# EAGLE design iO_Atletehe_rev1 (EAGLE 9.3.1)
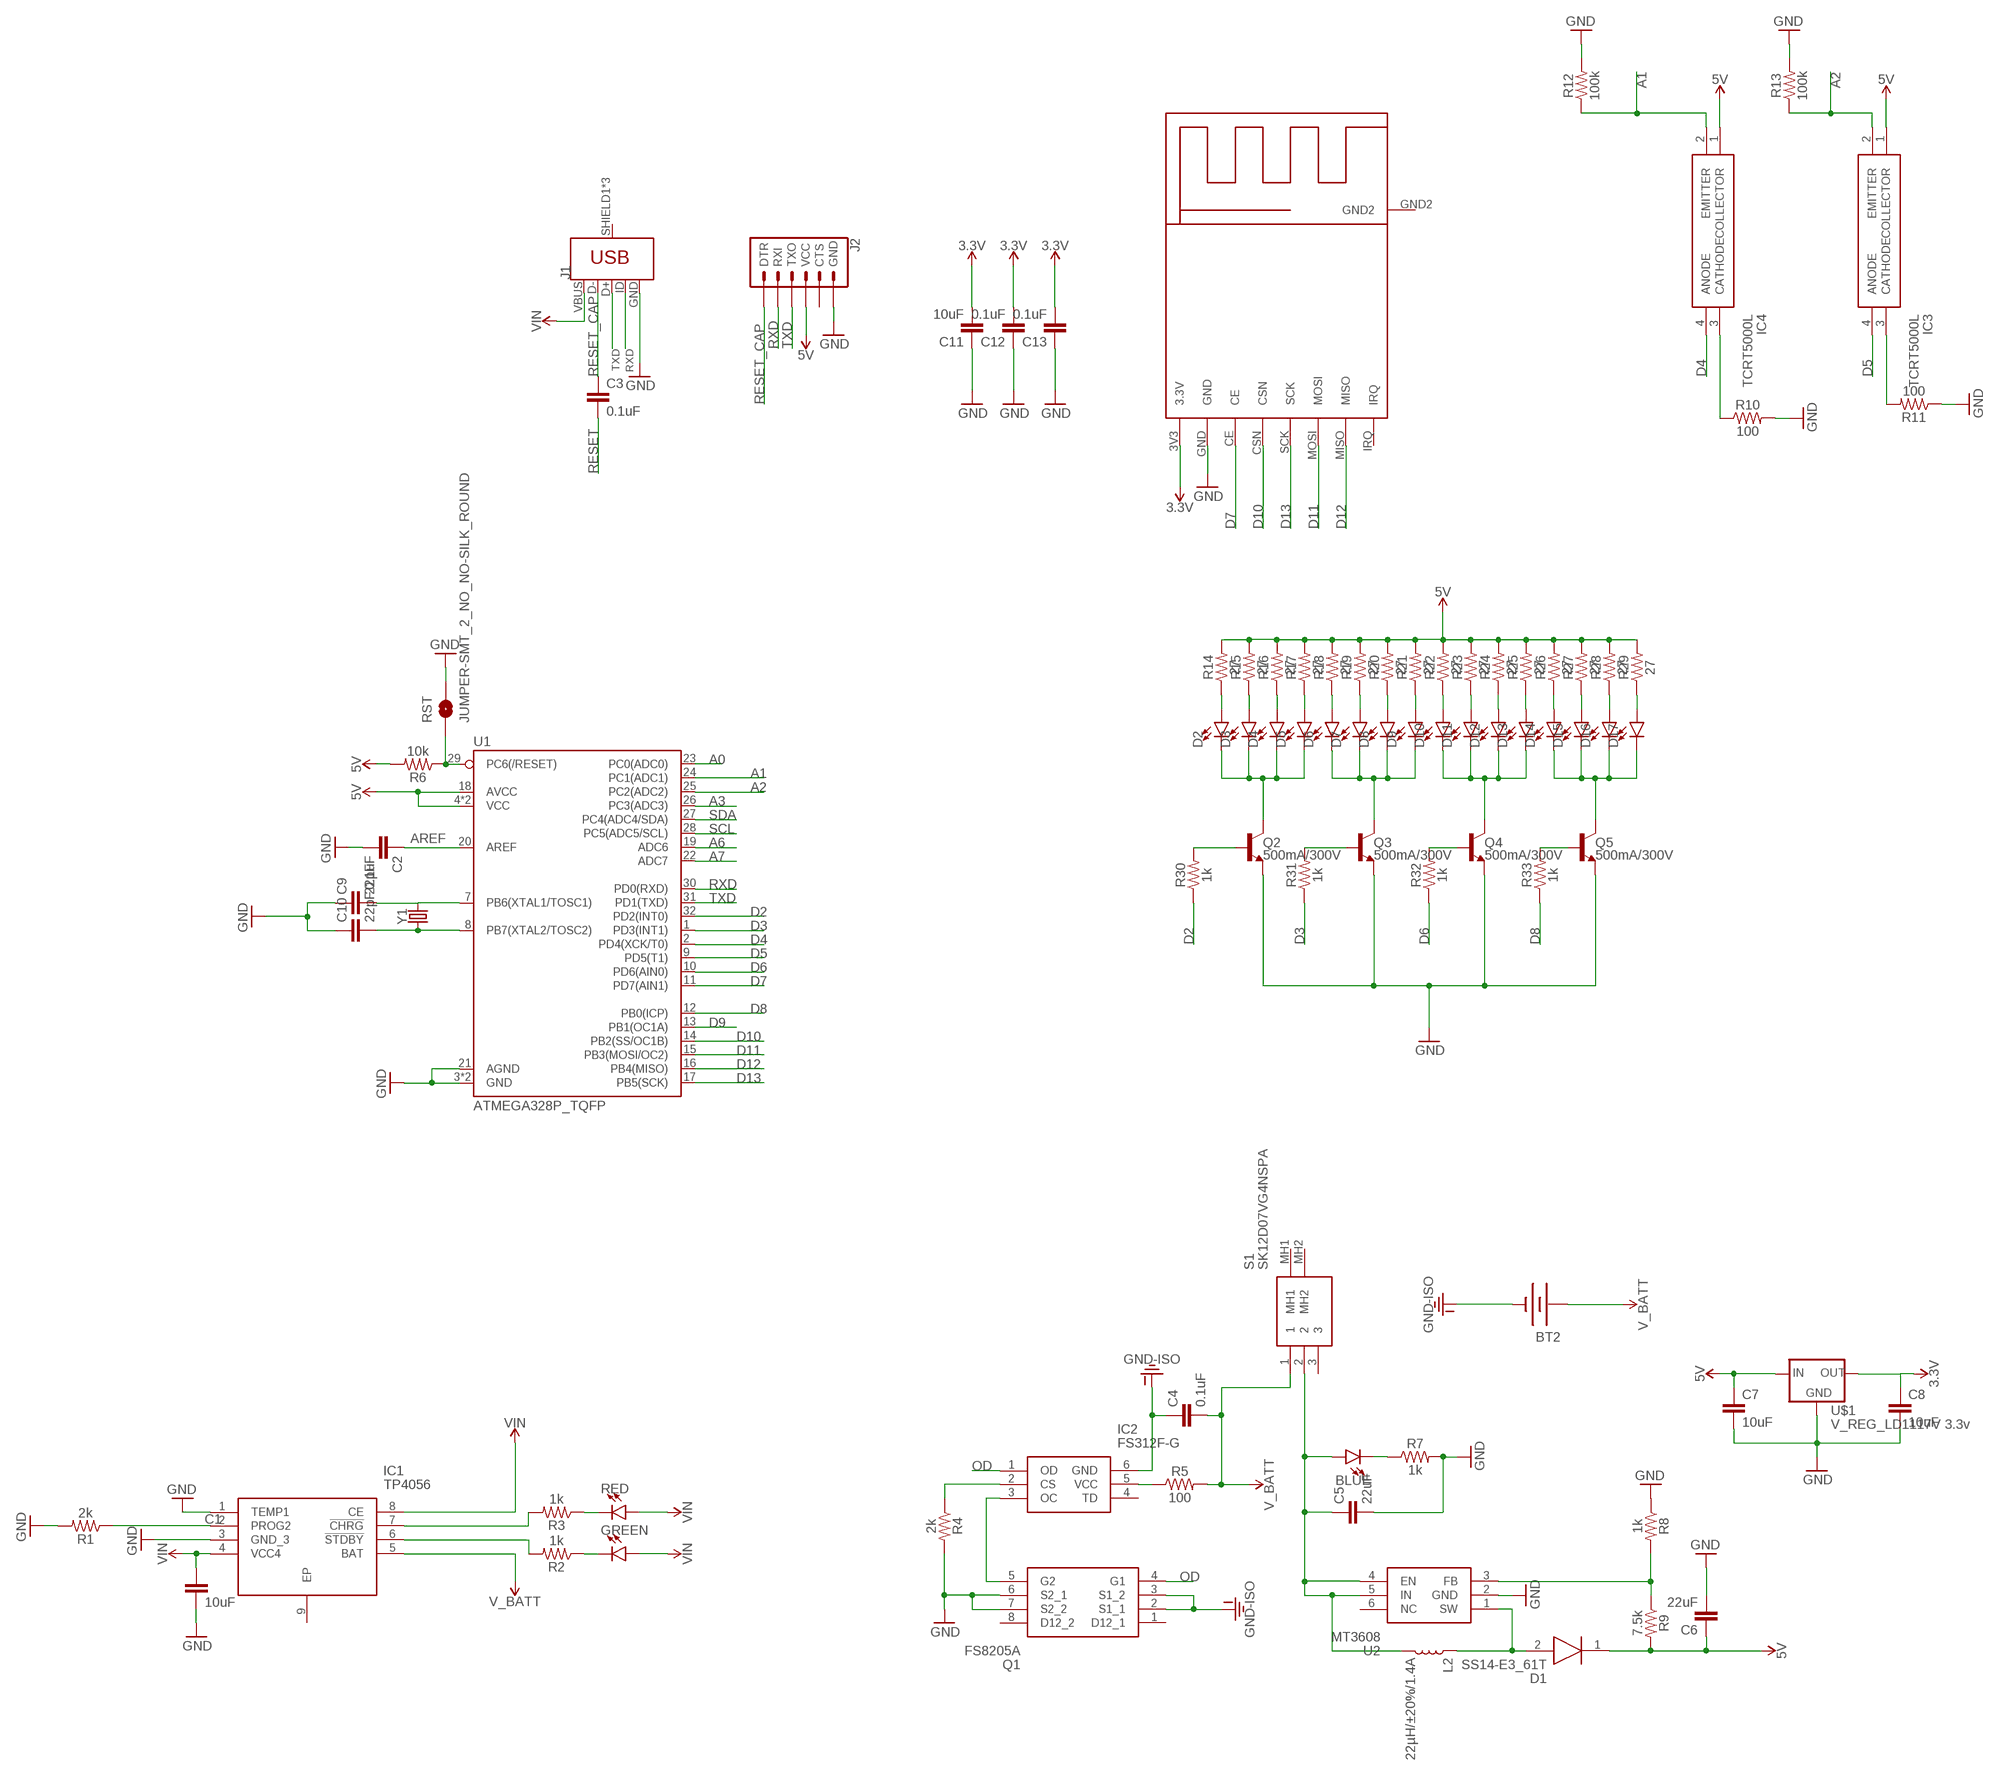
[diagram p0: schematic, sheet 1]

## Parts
BLUE  LED0603  [LED-0603]
BT2  BATTERY1100  [LIPO-1100MAH]
C1  10uF  10UF-0603-6.3V-20%  [0603]
C2  0.1uF  0.1UF-0603-25V-5%  [0603]
C3  0.1uF  0.1UF-0603-25V-5%  [0603]
C4  0.1uF  0.1UF-0603-25V-5%  [0603]
C5  22uF  10UF-0603-6.3V-20%  [0603]
C6  22uF  10UF-0603-6.3V-20%  [0603]
C7  10uF  10UF-0603-6.3V-20%  [0603]
C8  10uF  10UF-0603-6.3V-20%  [0603]
C9  22pF  22PF-0603-50V-5%  [0603]
C10  22pF  22PF-0603-50V-5%  [0603]
C11  10uF  10UF-0603-6.3V-20%  [0603]
C12  0.1uF  0.1UF-0603-25V-5%  [0603]
C13  0.1uF  0.1UF-0603-25V-5%  [0603]
D1  SS14-E3_61T  [DIOM5127X229N]
D2  LED5MM  [LED_5MM]
D3  LED5MM  [LED_5MM]
D4  LED5MM  [LED_5MM]
D5  LED5MM  [LED_5MM]
D6  LED5MM  [LED_5MM]
D7  LED5MM  [LED_5MM]
D8  LED5MM  [LED_5MM]
D9  LED5MM  [LED_5MM]
D10  LED5MM  [LED_5MM]
D11  LED5MM  [LED_5MM]
D12  LED5MM  [LED_5MM]
D13  LED5MM  [LED_5MM]
D14  LED5MM  [LED_5MM]
D15  LED5MM  [LED_5MM]
D16  LED5MM  [LED_5MM]
D17  LED5MM  [LED_5MM]
GREEN  LED0603  [LED-0603]
IC1  TP4056  [SOIC127P600X175-9N]
IC2  FS312F-G  [SOT95P280X145-6N]
IC3  TCRT5000L  [TCRT5000L]
IC4  TCRT5000L  [TCRT5000L]
J1  USB_MICRO-B_FEMALE-SMT  [USB-B-MICRO-SMD]
J2  6_PIN_SERIAL_TARGETPTH-KIT  [1X06-KIT]
L2  22µH/±20%/1.4A  INDUCTOR-SRN6045-33UH  [SRN6045]
Q1  FS8205A  [SOP65P640X120-8N]
Q2  500mA/300V  TRANS_NPN-MMBTA42  [SOT23-3]
Q3  500mA/300V  TRANS_NPN-MMBTA42  [SOT23-3]
Q4  500mA/300V  TRANS_NPN-MMBTA42  [SOT23-3]
Q5  500mA/300V  TRANS_NPN-MMBTA42  [SOT23-3]
R1  2k  10KOHM-0603-1/10W-1%  [0603]
R2  1k  10KOHM-0603-1/10W-1%  [0603]
R3  1k  10KOHM-0603-1/10W-1%  [0603]
R4  2k  10KOHM-0603-1/10W-1%  [0603]
R5  100  10KOHM-0603-1/10W-1%  [0603]
R6  10k  10KOHM-0603-1/10W-1%  [0603]
R7  1k  10KOHM-0603-1/10W-1%  [0603]
R8  1k  10KOHM-0603-1/10W-1%  [0603]
R9  7.5k  10KOHM-0603-1/10W-1%  [0603]
R10  100  10KOHM-0603-1/10W-1%  [0603]
R11  100  10KOHM-0603-1/10W-1%  [0603]
R12  100k  10KOHM-0603-1/10W-1%  [0603]
R13  100k  10KOHM-0603-1/10W-1%  [0603]
R14  27  27OHM-0603-1/10W-1%  [0603]
R15  27  27OHM-0603-1/10W-1%  [0603]
R16  27  27OHM-0603-1/10W-1%  [0603]
R17  27  27OHM-0603-1/10W-1%  [0603]
R18  27  27OHM-0603-1/10W-1%  [0603]
R19  27  27OHM-0603-1/10W-1%  [0603]
R20  27  27OHM-0603-1/10W-1%  [0603]
R21  27  27OHM-0603-1/10W-1%  [0603]
R22  27  27OHM-0603-1/10W-1%  [0603]
R23  27  27OHM-0603-1/10W-1%  [0603]
R24  27  27OHM-0603-1/10W-1%  [0603]
R25  27  27OHM-0603-1/10W-1%  [0603]
R26  27  27OHM-0603-1/10W-1%  [0603]
R27  27  27OHM-0603-1/10W-1%  [0603]
R28  27  27OHM-0603-1/10W-1%  [0603]
R29  27  27OHM-0603-1/10W-1%  [0603]
R30  1k  1KOHM-0603-1/10W-1%  [0603]
R31  1k  1KOHM-0603-1/10W-1%  [0603]
R32  1k  1KOHM-0603-1/10W-1%  [0603]
R33  1k  1KOHM-0603-1/10W-1%  [0603]
RED  LED0603  [LED-0603]
RST  JUMPER-SMT_2_NO_NO-SILK_ROUND  [SMT-JUMPER_2_NO_NO-SILK_ROUND]
S1  SK12D07VG4NSPA  [SK12D07VG4NSPA]
U1  ATMEGA328P_TQFP  [TQFP32-08]
U2  MT3608  [SOT95P280X145-6N]
U$1  V_REG_LD1117V 3.3v  V_REG_LD1117VXXLD1117-SMD  [SOT223]
U$2  NRF24MINI  [NRF24MINI]
Y1  CRYSTALSMD-HC49UP  [HC49UP]

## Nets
3.3V: C8.1 C11.2 C12.2 C13.2 U$1.2(OUT) U$2.3V3(3.3V)
5V: C6.1 C7.1 D1.1(K) IC3.1(COLLECTOR) IC4.1(COLLECTOR) J2.4(VCC) R6.2 R9.2 R14.2 R15.2 R16.2 R17.2 R18.2 R19.2 R20.2 R21.2 R22.2 R23.2 R24.2 R25.2 R26.2 R27.2 R28.2 R29.2 U1.4(VCC) U1.6(VCC) U1.18(AVCC) U$1.3(IN)
A0: U1.23(PC0(ADC0))
A1: IC4.2(EMITTER) R12.1 U1.24(PC1(ADC1))
A2: IC3.2(EMITTER) R13.1 U1.25(PC2(ADC2))
A3: U1.26(PC3(ADC3))
A6: U1.19(ADC6)
A7: U1.22(ADC7)
AREF: C2.1 U1.20(AREF)
D2: R30.1 U1.32(PD2(INT0))
D3: R31.1 U1.1(PD3(INT1))
D4: IC4.4(ANODE) U1.2(PD4(XCK/T0))
D5: IC3.4(ANODE) U1.9(PD5(T1))
D6: R32.1 U1.10(PD6(AIN0))
D7: U1.11(PD7(AIN1)) U$2.CE
D8: R33.1 U1.12(PB0(ICP))
D9: U1.13(PB1(OC1A))
D10: U1.14(PB2(SS/OC1B)) U$2.CSN
D11: U1.15(PB3(MOSI/OC2)) U$2.MOSI
D12: U1.16(PB4(MISO)) U$2.MISO
D13: U1.17(PB5(SCK)) U$2.SCK
GND [power]: C1.2 C2.2 C5.2 C6.2 C7.2 C8.2 C9.1 C10.1 C11.1 C12.1 C13.1 IC1.1(TEMP1) IC1.3(GND_3) J1.GND J2.6(GND) Q1.6(S2_1) Q1.7(S2_2) Q2.2(E) Q3.2(E) Q4.2(E) Q5.2(E) R1.2 R4.2 R7.2 R8.1 R10.2 R11.1 R12.2 R13.2 RST.2 U1.3(GND) U1.5(GND) U1.21(AGND) U2.2(GND) U$1.1(GND) U$2.GND
GND-ISO: BT2.- C4.1 IC2.6(GND) Q1.2(S1_1) Q1.3(S1_2)
N$1: IC2.3(OC) Q1.5(G2)
N$2: BLUE.C R7.1
N$3: IC1.2(PROG2) R1.1
N$4: GREEN.C R2.1
N$5: R3.1 RED.C
N$6: IC1.6(!STDBY) R2.2
N$7: IC1.7(!CHRG) R3.2
N$8: IC2.2(CS) R4.1
N$9: IC2.5(VCC) R5.1
N$10: C9.2 U1.7(PB6(XTAL1/TOSC1)) Y1.2
N$11: C10.2 U1.8(PB7(XTAL2/TOSC2)) Y1.1
N$12: D1.2(A) L2.1 U2.1(SW)
N$13: R8.2 R9.1 U2.3(FB)
N$14: BLUE.A C5.1 L2.2 S1.2 U2.4(EN) U2.5(IN)
N$15: IC4.3(CATHODE) R10.1
N$16: D2.A R14.1
N$17: IC3.3(CATHODE) R11.2
N$18: D3.A R15.1
N$19: D4.A R16.1
N$20: D5.A R17.1
N$21: D6.A R18.1
N$22: D7.A R19.1
N$23: D8.A R20.1
N$24: D9.A R21.1
N$25: D10.A R22.1
N$26: D11.A R23.1
N$27: D14.A R26.1
N$28: D13.A R25.1
N$29: D12.A R24.1
N$30: D15.A R27.1
N$31: D16.A R28.1
N$32: D17.A R29.1
N$34: D2.K(C) D3.K(C) D4.K(C) D5.K(C) Q2.3(C)
N$35: D6.K(C) D7.K(C) D8.K(C) D9.K(C) Q3.3(C)
N$36: D10.K(C) D11.K(C) D12.K(C) D13.K(C) Q4.3(C)
N$37: D14.K(C) D15.K(C) D16.K(C) D17.K(C) Q5.3(C)
N$38: Q2.1(B) R30.2
N$39: Q3.1(B) R31.2
N$40: Q4.1(B) R32.2
N$41: Q5.1(B) R33.2
OD: IC2.1(OD) Q1.4(G1)
RESET: C3.2 R6.1 RST.1 U1.29(PC6(/RESET))
RESET_CAP: C3.1 J1.D- J2.1(DTR)
RXD: J1.ID J2.2(RXI) U1.30(PD0(RXD))
SCL: U1.28(PC5(ADC5/SCL))
SDA: U1.27(PC4(ADC4/SDA))
TXD: J1.D+ J2.3(TXO) U1.31(PD1(TXD))
V_BATT: BT2.+ C4.2 IC1.5(BAT) R5.2 S1.1
VIN: C1.1 GREEN.A IC1.4(VCC4) IC1.8(CE) J1.VBUS RED.A
Unconnected: IC1.9(EP) IC2.4(TD) J1.SHIELD1(SHIELD) J1.SHIELD2(SHIELD) J1.SHIELD3(SHIELD) J2.5(CTS) Q1.1(D12_1) Q1.8(D12_2) S1.3 S1.MH1 S1.MH2 U2.6(NC) U$2.GND2 U$2.IRQ

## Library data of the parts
BLUE D2-D17 GREEN RED = SparkFun-LED:LED: LED (Generic)
BT2 = SparkFun-Retired:BATTERY: Battery - Single Cell
C1 C7 C8 C11 = SparkFun-Capacitors:10UF: 10.0µF ceramic capacitors; PROD_ID: CAP-11015
C2-C4 C12 C13 = SparkFun-Capacitors:0.1UF: 0.1µF ceramic capacitors; PROD_ID: CAP-08604
C5 C6 = SparkFun-Capacitors:10UF: 10.0µF ceramic capacitors; PROD_ID: CAP-11015; VALUE: 10uF
C9 C10 = SparkFun-Capacitors:22PF: 22pF ceramic capacitors; PROD_ID: CAP-07876
D1 = SS14-E3_61T:SS14-E3_61T: Schottky Diode 1A 40V 0.5Vf DO-214AC Vishay SS14-E3/61T, SMT Schottky Diode, 40V 1A, 2-Pin DO-214AC; ALLIED_NUMBER: 70217666; ALLIED_PRICE-STOCK: https://www.alliedelec.com/general-semiconductor-vishay-ss14-e3-61t/70217666/; DESCRIPTION: Schottky Diode 1A 40V 0.5Vf DO-214AC Vishay SS14-E3/61T, SMT Schottky Diode, 40V 1A, 2-Pin DO-214AC; HEIGHT: 2.29mm; MANUFACTURER_NAME: Vishay; MANUFACTURER_PART_NUMBER: SS14-E3/61T; MOUSER_PART_NUMBER: 625-SS14-E3; MOUSER_PRICE-STOCK: https://www.mouser.com/Search/Refine.aspx?Keyword=625-SS14-E3; RS_PART_NUMBER: 6387915P; RS_PRICE-STOCK: http://uk.rs-online.com/web/p/products/6387915P
IC1 = TP4056:TP4056: 1A Standalone Linear Li-lon Battery Charger, SOP-8 Source: Datasheet; DESCRIPTION: 1A Standalone Linear Li-lon Battery Charger, SOP-8; HEIGHT: 1.75mm; MANUFACTURER_NAME: NanJing Top Power; MANUFACTURER_PART_NUMBER: TP4056
IC2 = FS312F-G:FS312F-G: One Cell Lithium-ion/Polymer Battery Protection IC Source: Datasheet; DESCRIPTION: One Cell Lithium-ion/Polymer Battery Protection IC; HEIGHT: 1.45mm; MANUFACTURER_NAME: Fortune Semiconductor Corporation; MANUFACTURER_PART_NUMBER: FS312F-G
IC3 IC4 = TCRT5000L:TCRT5000L: Photointerrupter Reflective Phototransi Vishay TCRT5000L PCB Through Hole Reflective Optical Sensor, Transistor Output 2, Leaded Package Source: Datasheet; ALLIED_NUMBER: 70617350; ALLIED_PRICE-STOCK: http://www.alliedelec.com/siliconix-vishay-tcrt5000l/70617350/; DESCRIPTION: Photointerrupter Reflective Phototransi Vishay TCRT5000L PCB Through Hole Reflective Optical Sensor, Transistor Output 2, Leaded Package; HEIGHT: mm; MANUFACTURER_NAME: Vishay; MANUFACTURER_PART_NUMBER: TCRT5000L; MOUSER_PART_NUMBER: 782-TCRT5000L; MOUSER_PRICE-STOCK: https://www.mouser.com/Search/Refine.aspx?Keyword=782-TCRT5000L; RS_PART_NUMBER: 1451738; RS_PRICE-STOCK: http://uk.rs-online.com/web/p/products/1451738
J1 = SparkFun-Connectors:USB_MICRO-B: USB Type Micro-B Connector Male/female and PTH/SMT variants SparkFun Products: SparkFun microB USB Breakout SparkFun USB microB Plug Breakout SparkFun ESP8266 Thing; PROD_ID: CONN-11752
J2 = SparkFun-Connectors:6_PIN_SERIAL_TARGET: 6-pin header connection for use with the "FTDI BASIC" pinout - TARGET SIDE. Also known as "Arduino Serial Program Header". It is used to mate with our FTDI Basic serial programmers using the Arduino IDE. Note, this device has "TARGET" in the name. It is intended to be used on a design that contains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
L2 = SparkFun-Coils:INDUCTOR: Inductors; PROD_ID: NDUC-11627; VALUE: 33µH/±20%/1.4A
Q1 = FS8205A:FS8205A: dual n-channel enhancement mode power MOFSET Source: Datasheet; DESCRIPTION: dual n-channel enhancement mode power MOFSET; HEIGHT: 1.2mm; MANUFACTURER_NAME: SII Semiconductor; MANUFACTURER_PART_NUMBER: FS8205A
Q2-Q5 = SparkFun-DiscreteSemi:TRANS_NPN: NPN transistor Current controlled devices typically used to amplify current or used as a switch. BC547 - COM-08928 (TO-92 45V 100mA) (1.Collector 2.Base 3.Emitter) 2N3904 - COM-00521 (TO-92 40V 200mA) (1.Emitter 2.Base 3.Collector) P2N2222A - COM-12852 (TO-92 40V 600mA) (1.Collector 2.Base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; PROD_ID: TRANS-09116
R1-R5 R7-R13 = SparkFun-Resistors:10KOHM: 10kΩ resistor; PROD_ID: RES-00824; VALUE: 10k
R6 = SparkFun-Resistors:10KOHM: 10kΩ resistor; PROD_ID: RES-00824
R14-R29 = SparkFun-Resistors:27OHM: 27Ω resistor; PROD_ID: RES-09334
R30-R33 = SparkFun-Resistors:1KOHM: 1kΩ resistor; PROD_ID: RES-07856
RST = SparkFun-Jumpers:JUMPER-SMT_2_NO: Normally open jumper
S1 = SK12D07VG4NSPA:SK12D07VG4NSPA: Slide Switches Miniature Slide Switch Source: Datasheet; DESCRIPTION: Slide Switches Miniature Slide Switch; HEIGHT: 4.7mm; MANUFACTURER_NAME: C & K COMPONENTS; MANUFACTURER_PART_NUMBER: SK12D07VG4NSPA; MOUSER_PART_NUMBER: 611-SK12D07VG4NSPA; MOUSER_PRICE-STOCK: https://www.mouser.com/Search/Refine.aspx?Keyword=611-SK12D07VG4NSPA
U1 = SparkFun-IC-Microcontroller:ATMEGA328P_TQFP: Popular 328P in QFP Storefront component: ATmega328 - TQFP (COM-13448) Datasheet SparkFun Products SparkFun RedBoard - Programmed with Arduino (DEV-12757) Arduino Pro Mini 328 - 5V/16MHz (DEV-11113) Arduino Pro Mini 328 - 3.3V/8MHz (DEV-11114) SparkFun OpenLog (DEV-13712) SparkFun MicroView - OLED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; PROD_ID: IC-09069; SPICEPREFIX: X
U2 = MT3608:MT3608: High Efficiency 1.2MHz 2A Step Up Converter Source: Datasheet; DESCRIPTION: High Efficiency 1.2MHz 2A Step Up Converter; HEIGHT: 1.45mm; MANUFACTURER_NAME: Aerosemi; MANUFACTURER_PART_NUMBER: MT3608
U$1 = SparkFun-IC-Power:V_REG_LD1117VXX: LD1117VXX voltage regulator. We carry the 3.3V version (COM-00526) in TO-220 package.; PROD_ID: VREG-13917
U$2 = nrf24mini:NRF24MINI
Y1 = SparkFun-Clocks:CRYSTAL: Crystals (Generic)

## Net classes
1 power: width 0.305 mm

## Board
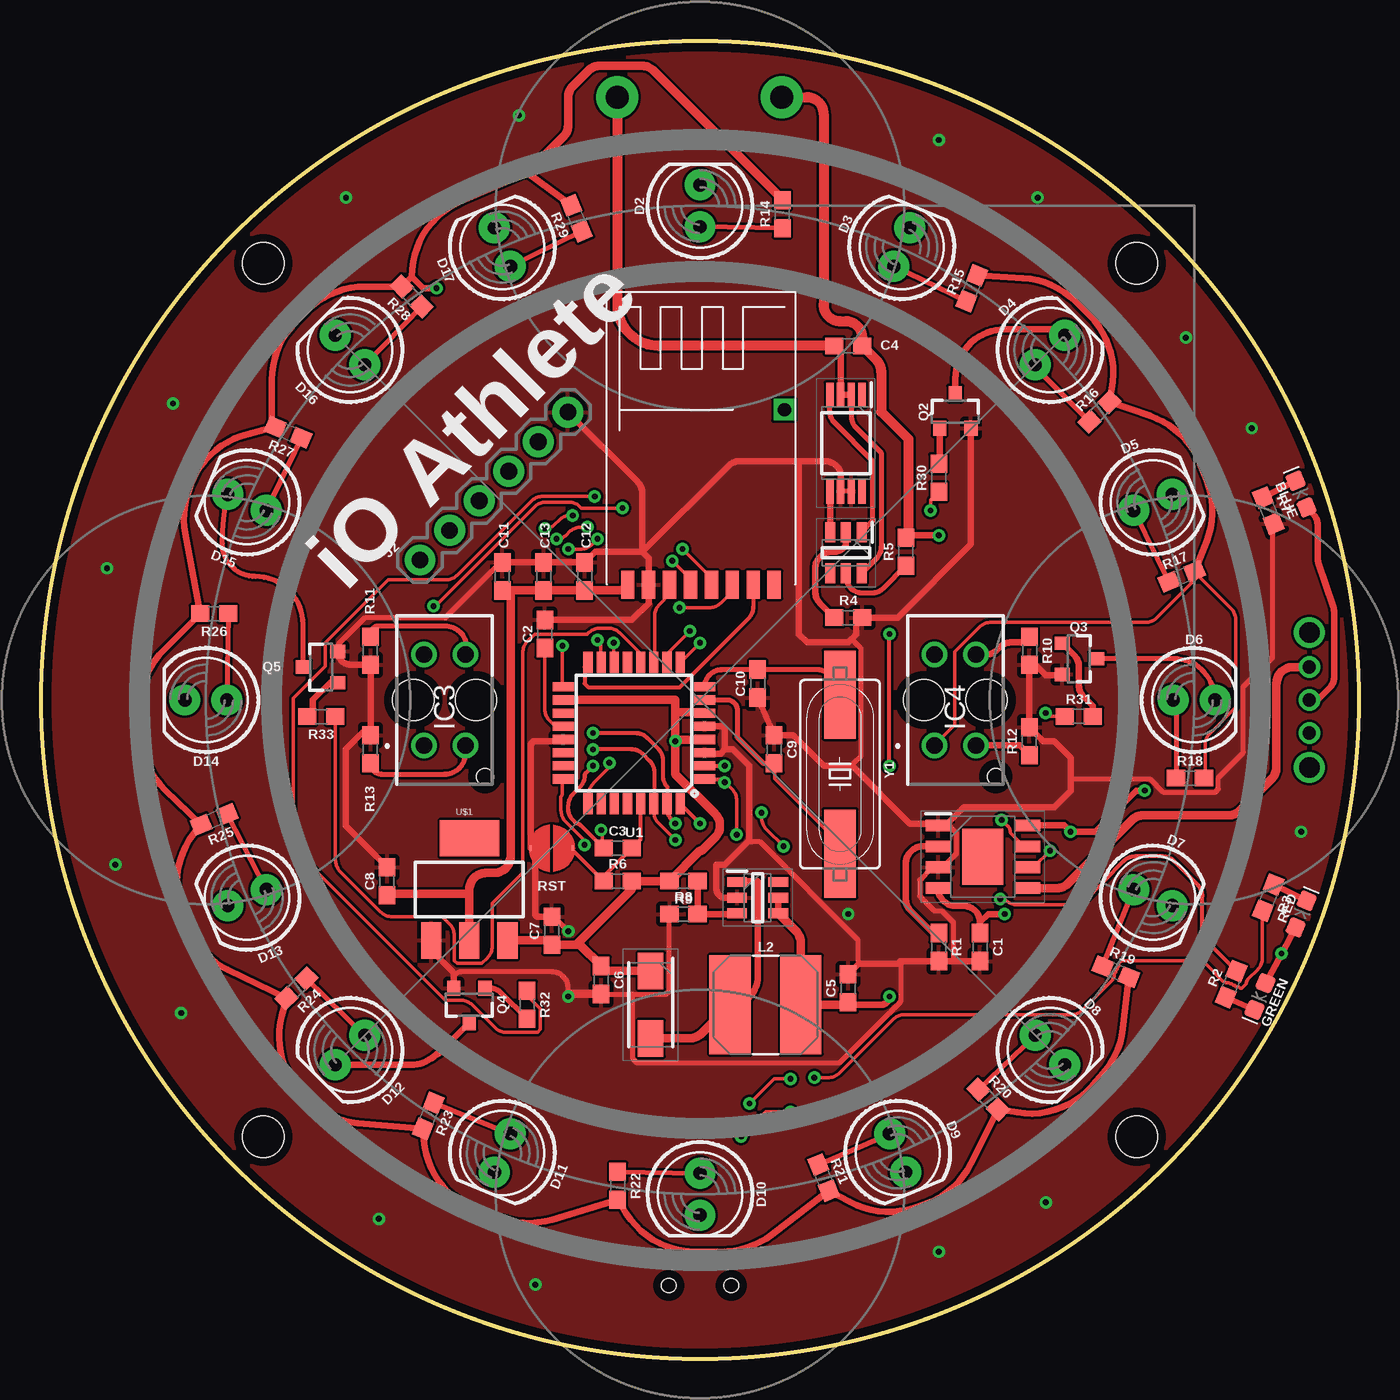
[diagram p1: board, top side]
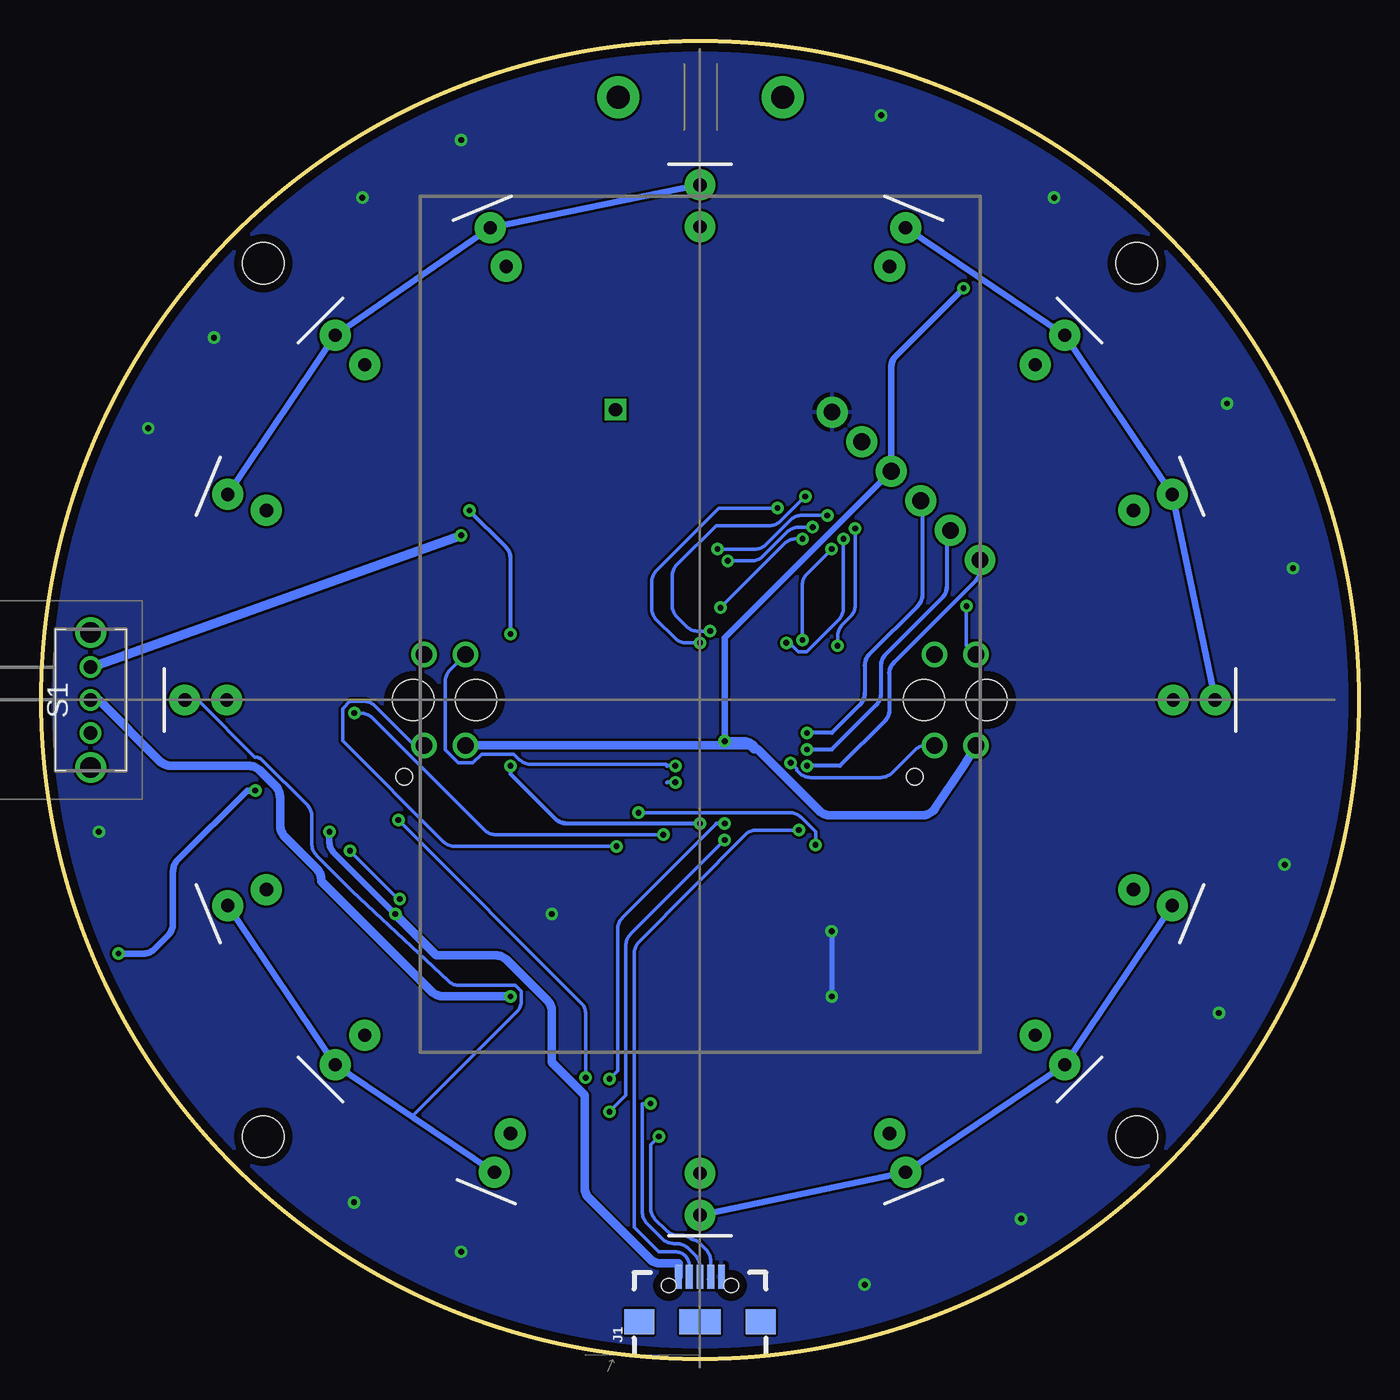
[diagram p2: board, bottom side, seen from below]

Size 80 x 80 mm. Coordinates in mm from the lower left corner, seen from the top.
Outline: circle at 40,40 radius 40
Copper layers (1*16): Top 0.035mm / dielectric 1.5mm / Bottom 0.035mm
Design rules "default *": minimum track width 8mil, minimum drill 0.35mm, track to track 6mil, track to pad 6mil, pad to pad 6mil, via to via 6mil, smd to smd 6mil, copper to edge 20mil, drill to drill 6mil, minimum pad ring 10mil, minimum via ring 8mil, stop-mask expansion 4mil, vias tented up to drill 0mil, thermal gap 10mil
Holes 2.5 mm at 13.48,13.48 66.52,66.52 66.52,13.48 13.48,66.52

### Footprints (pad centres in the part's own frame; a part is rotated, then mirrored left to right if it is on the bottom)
LED-0603 = smd 1 x 1: A -0.877,0; C 0.877,0
LIPO-1100MAH = drill 1.397 pad 2.54: + -5,32; - 5,32
0603 = smd 1.1 x 1: 1 -0.85,0; 2 0.85,0
DIOM5127X229N = smd 2.2 x 1.55: 1 -2.05,0; 2 2.05,0
LED_5MM = drill 0.813 pad 1.88: A -1.27,0; K 1.27,0
SOIC127P600X175-9N = smd 1.525 x 0.7: 1 -2.712,1.905; 2 -2.712,0.635; 3 -2.712,-0.635; 4 -2.712,-1.905; 5 2.712,-1.905; 6 2.712,-0.635; 7 2.712,0.635; 8 2.712,1.905 | smd 2.513 x 3.402: 9 0,0
SOT95P280X145-6N = smd 1.2 x 0.6: 1 -1.25,0.95; 2 -1.25,0; 3 -1.25,-0.95; 4 1.25,-0.95; 5 1.25,0; 6 1.25,0.95
TCRT5000L = drill 1 pad 1.55: 1 -2.75,1.27; 2 -2.75,-1.27; 3 2.75,-1.27; 4 2.75,1.27 | hole 2.5: 0,1.9; 0,-1.9 | hole 1: -4.65,-2.45
USB-B-MICRO-SMD = smd 1.45 x 0.4: D+ 2.725,0; D- 2.725,0.65; GND 2.725,-1.3; ID 2.725,-0.65; VBUS 2.725,1.3 | smd 1.5 x 1.8: SHIELD1 0,3.685; SHIELD2 0,-3.685 | smd 1.5 x 2.5: SHIELD3 0,0 | hole 0.85: 2.2,1.9; 2.2,-1.9
1X06-KIT = drill 1.016 pad 1.88: 1 0,0; 2 2.54,0; 3 5.08,0; 4 7.62,0; 5 10.16,0; 6 12.7,0
SRN6045 = smd 2.5 x 6: 1 -2.175,0; 2 2.125,0
SOP65P640X120-8N = smd 1.475 x 0.45: 1 -2.938,0.975; 2 -2.938,0.325; 3 -2.938,-0.325; 4 -2.938,-0.975; 5 2.938,-0.975; 6 2.938,-0.325; 7 2.938,0.325; 8 2.938,0.975
SOT23-3 = smd 0.8 x 0.9: 1 -0.95,-1; 2 0.95,-1; 3 0,1.1
SMT-JUMPER_2_NO_NO-SILK_ROUND = smd 0.152 x 0.305: 1 -1.27,0; 2 1.27,0
SK12D07VG4NSPA = drill 0.8 pad 1.3: 1 0,0; 2 2,0; 3 4,0 | drill 1.25 pad 1.875: MH1 -2.1,0; MH2 6.1,0
TQFP32-08 = smd 1.27 x 0.559: 1 -4.293,2.8; 2 -4.293,2; 3 -4.293,1.2; 4 -4.293,0.4; 5 -4.293,-0.4; 6 -4.293,-1.2; 7 -4.293,-2; 8 -4.293,-2.8; 17 4.293,-2.8; 18 4.293,-2; 19 4.293,-1.2; 20 4.293,-0.4; 21 4.293,0.4; 22 4.293,1.2; 23 4.293,2; 24 4.293,2.8 | smd 0.559 x 1.27: 9 -2.8,-4.293; 10 -2,-4.293; 11 -1.2,-4.293; 12 -0.4,-4.293; 13 0.4,-4.293; 14 1.2,-4.293; 15 2,-4.293; 16 2.8,-4.293; 25 2.8,4.293; 26 2,4.293; 27 1.2,4.293; 28 0.4,4.293; 29 -0.4,4.293; 30 -1.2,4.293; 31 -2,4.293; 32 -2.8,4.293
SOT223 = smd 1.219 x 2.235: 1 -2.311,-3.099; 2 0,-3.099; 3 2.311,-3.099 | smd 3.6 x 2.2: 4 0,3.099
NRF24MINI = smd 1.676 x 0.813: 3V3 0,8.89; CE 0,6.35; CSN 0,5.08; GND 0,7.62; IRQ 0,0; MISO 0,1.27; MOSI 0,2.54; SCK 0,3.81 | drill 0.8 square: GND2 10.625,-0.625
HC49UP = smd 5.334 x 1.93: 1 -4.826,0; 2 4.826,0

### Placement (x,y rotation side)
BLUE  76.5,52.5 112.5 top
BT2  39.97,44.6 0 bottom
C1  57,25 270 top
C2  30.58,44.01 90 top
C3  35,31 0 top
C4  49,61.5 0 top
C5  49,22.5 90 top
C6  34,23 270 top
C7  31,26 90 top
C8  21,29 90 top
C9  44.5,37 270 top
C10  43.5,41 90 top
C11  28,47.5 270 top
C12  33,47.5 270 top
C13  30.5,47.5 270 top
D1  37,21.5 270 top
D2  40,70 90 top
D3  52.25,67.5 67.5 top
D4  61.25,61.25 45 top
D5  67.5,52 22.5 top
D6  70,40 0 top
D7  67.5,28 337.5 top
D8  61.25,18.75 315 top
D9  52,12.5 292.5 top
D10  40,10 270 top
D11  28,12.5 247.5 top
D12  18.75,18.75 225 top
D13  12.5,28 202.5 top
D14  10,40 180 top
D15  12.5,52 157.5 top
D16  18.75,61.25 135 top
D17  28,67.5 112.5 top
GREEN  74,22 247.5 top
IC1  57.17,30.48 0 top
IC2  48.86,48.94 270 top
IC3  24.5,40 90 top
IC4  55.5,40 90 top
J1  40,2.25 90 bottom
J2  23,48.5 45 top
L2  44,21.5 0 top
Q1  48.86,55.6 270 top
Q2  55.5,57.5 0 top
Q3  63,42.5 270 top
Q4  26,21.5 180 top
Q5  17,42 90 top
R1  54.5,25 270 top
R2  72.25,22.75 67.5 top
R3  74.5,28 247.5 top
R4  49,45 0 top
R5  52.5,49 90 top
R6  35,29 0 top
R7  74.5,51.5 292.5 top
R8  39,27 0 top
R9  39,29 180 top
R10  60,43 270 top
R11  20,43 90 top
R12  60,37.5 90 top
R13  20,37 90 top
R14  45,69.5 90 top
R15  56.5,65 67.5 top
R16  64.25,57.5 45 top
R17  69.25,47.5 22.5 top
R18  69.75,35.25 0 top
R19  65.25,23.5 337.5 top
R20  57.5,15.75 315 top
R21  47.5,11 292.5 top
R22  35,10.5 270 top
R23  23.5,14.75 247.5 top
R24  15.5,22.5 225 top
R25  10.5,32.75 202.5 top
R26  10.5,45.25 180 top
R27  15,56.25 157.5 top
R28  22.5,64.5 135 top
R29  32.5,69.25 112.5 top
R30  54.5,53.5 90 top
R31  63,39 0 top
R32  29.5,21.5 270 top
R33  17,39 180 top
RED  76.5,27 67.5 top
RST  31,31 180 top
S1  77,42 270 bottom
U1  36,38 180 top
U2  43.5,28 0 top
U$1  26,28.5 0 top
U$2  44.5,47 90 top
Y1  48.5,35.5 270 top

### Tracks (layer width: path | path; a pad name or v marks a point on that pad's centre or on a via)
3.3V
  Top 0.508: U$2.3V3 35.26,46.65 C12.2 C13.2 28.5,46.65 | 28.5,46.65 C11.2 | U$1.2 26,28.25 | 26,28.25 21,28.25 C8.1 | 26,28.25 26,28.5 arc-90 27,29.5 27.5,29.5 arc90 28.5,30.5 28.5,46.65
5V  (via drill 0.35)
  Top 0.203: R18.2 70.67,35.29 70.67,37.28 arc-45 70.97,37.99 72.54,39.56 72.54,44.84 arc45 72.25,45.54 70.14,47.65 R17.2 70.23,47.47 67.77,45.01 arc-45 67.06,44.72 57.67,44.72 arc45 56.96,44.42 55.47,42.94 55.47,38.49 54.32,37.34 IC4.1 | 44.98,70.41 R14.2 | 29.52,72.19 29.5,72
  Top 0.406: 22.5,65.7 R28.2 19.67,65.1 arc45 16.14,63.64 15.46,62.96 arc45 14,59.43 14,56.79 R27.2 12.53,56.15 arc55 9.08,53.06 8.99,52.8 arc31 8.75,50.14 R26.2 7.46,43.06 arc45 6,39.53 6,38.13 arc46 7.53,34.52 R25.2 9.54,32.23 arc62 8.54,27.16 8.8,26.41 arc44 11.33,23.62 R24.2 14.62,20.84 arc52 15.45,16.56 15.66,16.29 arc48 19.23,14.31 R23.2 23.23,13.29 arc67 26.63,8.96 28,8.5 arc35 31.02,8.46 R22.2 35.53,8.82 arc58 39.75,6.5 41.3,6.5 arc38 44.35,7.54 R21.2 49.1,9.53 arc47 53.05,9.18 53.55,9.35 arc45 56.43,11.84 R20.2 59.25,14.96 arc58 63.84,16.6 64.47,17.33 arc35 65.68,20.05 R19.2 | 22.5,65.7 22.5,65.7 arc-67 25.53,70.3 29.5,72 R29.2 | R15.2 59.61,65.61 arc-42 62.84,64.16 63.63,63.37 arc-56 65,58.9 R16.2 67.34,57.24 arc-49 70.35,54.38 70.76,53.35 arc-44 70.76,49.65 R17.2 | v24,65 23.2,65 22.5,65.7
  Top 0.508: D1.1 34.3,23.55 C6.1 32.7,25.15 32.5,25.15 | U$1.3 30.75,25.4 C7.1 32.5,25.15 | 32.5,25.15 35.85,28.5 R6.2 R9.2 40,30.85 40.1,30.85 40.92,31.67 arc90 40.92,33.08 38.5,35.5 v38.5,37.5 38.5,37.6 | U1.18 38.5,40 38.5,39.25 | 38.5,39.25 40.29,39.25 U1.6 | 38.5,37.6 38.5,39.25 | 38.5,37.6 U1.4 | 29.5,72 31.71,74.21 arc45 32,74.91 32,76.59 arc-45 32.29,77.29 33.21,78.21 arc-45 33.91,78.5 36.48,78.5 arc-45 37.19,78.21 44.98,70.41
  Bottom 0.406: v38.5,37.5 38.5,43.78 J2.4 28.39,60.2 arc45 28.09,60.91 v24,65
  Bottom 0.508: IC3.1 24,36 25.7,33.45 arc56 26.54,33 32.09,33 arc45 32.79,33.29 36.5,37 | 36.75,37.25 37,37.25 | 37,37.25 IC4.1 | 37,37.25 36.75,37 36.5,37 | v38.5,37.5 37.41,37.5 arc45 36.71,37.21 36.5,37
A1  (via drill 0.35)
  Top 0.203: v32.98,31.2 32.98,31.47 31.85,32.6 arc-45 31.56,33.31 31.56,34.14 arc45 31.65,34.35 31.65,35.12 U1.24 | v45.07,31.11 44.03,32.16 arc-45 43.74,32.86 v43.74,33.16
  Top 0.406: R12.1 59.4,37.25 IC4.2
  Bottom 0.203: v32.98,31.2 32.98,32 33.84,32.87 arc-45 34.55,33.16 v43.74,33.16 | v45.07,31.11 54.88,31.11 arc45 55.59,31.41 61.7,37.52 61.7,39.47 61.25,39.92 60.42,39.92 arc45 59.72,39.62 57.43,37.34 56.81,37.34 IC4.2
A2  (via drill 0.35)
  Top 0.203: v34.49,36.18 34.49,35.92 33.54,34.96 arc45 33.25,34.26 33.25,33.78 U1.25
  Top 0.305: R13.1 arc90 20.65,35.5 24.5,35.5 arc90 25.77,36.77 IC3.2
  Bottom 0.203: v34.49,36.18 34.14,35.83 34.14,35.74 33.99,35.59 arc-45 33.28,35.29 29.04,35.29 arc-45 28.33,35.59 26.96,36.96 arc45 26.26,37.25 IC3.2
AREF
  Top 0.203: C2.1 30.58,43.12 30.58,39.44 arc45 30.87,38.73 31.2,38.41 31.65,38.41 U1.20
D2  (via drill 0.35)
  Top 0.203: R30.1 54,52.15 v54,51.5
  Top 0.254: U1.32 v40,32.51 v40,32.5 | v51.5,36 v51.5,44
  Bottom 0.254: v40,32.5 48.09,32.5 arc45 48.79,32.79 51.5,35.5 v51.5,36 | v51.5,44 51.5,48.59 arc-45 51.79,49.29 v54,51.5
D3  (via drill 0.35)
  Top 0.203: v60.98,39.2 61.16,39.03 62.14,39.03 R31.1 | v42.23,31.83 42.23,33.9 arc45 41.94,34.61 41.6,34.94 v41.5,35
  Top 0.254: U1.1 41.3,35.2 v41.5,35
  Bottom 0.203: v60.98,39.2 60.6,39.2 arc45 59.89,38.91 53.1,32.12 arc-45 52.39,31.83 v42.23,31.83
  Bottom 0.254: v41.5,35 42,35
D4  (via drill 0.35)
  Top 0.254: U1.2 v41.5,36
  Bottom 0.203: 42,36 42.05,36.09 50.26,36.09 arc45 50.97,36.39 51.3,36.72 53.25,36.72 53.78,36.18 54.67,36.18 55.47,36.98 55.47,41.1 arc45 55.18,41.81 54.32,42.67 IC4.4
  Bottom 0.254: v41.5,36 42,36
D5  (via drill 0.35)
  Top 0.203: v40.01,43.47 38.85,42.32 U1.9 | v35.29,51.65 32.8,51.65 32.74,51.71 arc45 32.03,52.01 30.64,52.01 arc45 29.93,51.71 23.91,45.7 v23.82,45.7
  Bottom 0.203: v40.01,43.47 40.84,43.47 arc45 41.54,43.77 42.65,44.87 arc45 42.94,45.58 42.94,47.15 arc45 42.65,47.85 38.85,51.65 v35.29,51.65 | v23.82,45.7 23.82,43.29 23.29,42.76 IC3.4
D6  (via drill 0.35)
  Top 0.203: v33.6,52.36 30.46,52.36 arc45 29.75,52.07 25.27,47.59 arc-45 24.57,47.3 21.07,47.3 17.25,43.47 17.25,42.05 15.29,40.09 15.29,31.44 arc45 15.58,30.73 24.54,21.78 25.46,21.78 arc-45 26.16,21.49 27.53,20.12 arc45 28.24,19.82 30.14,19.82 30.32,20 30.32,21.25 29.52,22.05 29.52,22.31 R32.1 | v39.38,44.18 38.05,42.85 38.05,42.32 U1.10
  Bottom 0.203: v33.6,52.36 35.09,50.88 arc45 35.8,50.58 39.03,50.58 41.4,48.21 arc-45 41.69,47.5 41.69,45.75 arc-45 41.4,45.05 40.83,44.48 arc-45 40.12,44.18 v39.38,44.18
D7
  Top 0.203: U1.11 37.25,42.32 37.25,45.1 arc-45 37.54,45.81 38.14,46.41 38.14,46.94 U$2.CE
D8
  Top 0.203: R33.1 17.87,38.94 17.87,30.29 arc45 18.16,29.58 20.6,27.14 arc45 21.31,26.85 24.36,26.85 24.78,26.43 arc-45 25.07,25.72 25.07,24.18 25.25,24 26.76,24 27.09,24.33 arc45 27.38,25.04 27.38,27.65 29.25,29.52 29.25,42.88 arc-45 29.54,43.59 29.96,44.01 33.16,44.01 33.22,44.07 arc-45 33.93,44.36 34.44,44.36 arc-45 35.14,44.07 36.36,42.85 36.36,42.32 U1.12
D10  (via drill 0.35)
  Top 0.203: v34.76,43.47 34.76,42.32 U1.14 | v31.29,49.78 arc45 31.9,50.03 32.07,50.2 arc-45 32.77,50.49 v33.16,50.49 | v38.32,48.45 39.38,47.38 39.38,47.03 U$2.CSN
  Bottom 0.203: v34.76,43.47 34.58,43.47 34.05,42.94 33.52,42.94 31.59,44.87 arc-45 31.29,45.58 v31.29,49.78 | v38.32,48.45 36.86,48.45 arc-45 36.16,48.74 34.7,50.2 arc45 33.99,50.49 v33.16,50.49
D11  (via drill 0.35)
  Top 0.203: v33.78,43.65 33.96,43.47 33.96,42.32 U1.15 | v33.78,49.78 33.45,49.45 arc-45 32.74,49.16 v32,49.16 | v38.76,45.61 40.57,45.61 arc45 41.28,45.9 41.87,46.49 41.87,46.94 U$2.MOSI
  Bottom 0.203: v32,49.16 33.49,47.68 arc-45 33.78,46.97 v33.78,43.65 | v38.76,45.61 34.88,49.49 arc45 34.17,49.78 v33.78,49.78
D12
  Top 0.254: U$2.MISO 43.23,45.64 arc-45 42.94,44.94 38.75,40.75 33.25,40.75 33,41 33,42 33.2,42.2 U1.16
D13  (via drill 0.35)
  Top 0.203: v31.65,43.29 31.65,40.8 U1.17 | v30.58,50.41 arc45 31.19,50.66 31.44,50.91 arc-45 32.15,51.21 v32.27,51.21 | v38.94,49.16 40.63,47.47 40.63,47.03 U$2.SCK
  Bottom 0.203: v31.65,43.29 31.65,43.86 arc45 31.36,44.56 30.87,45.05 arc-45 30.58,45.75 v30.58,50.41 | v38.94,49.16 36.69,49.16 arc-45 35.98,49.45 34.52,50.91 arc45 33.81,51.21 v32.27,51.21
GND  (via drill 0.35)
  Top 0.305: Q1.7 Q1.6 | v32,22 32,22.5 arc90 31,23.5 25.5,23.5 arc90 25,23 25,22.55 arc90 Q4.2 | Q5.2 18.05,43.12 18.05,43.38 19.65,44.98 24.54,44.98 27.83,48.27 C11.1 | 35.92,22.14 34.23,22.14 C6.2 | 35.92,22.14 37.96,22.14 38.14,22.31 38.14,26.94 R8.1 | v32,25.96 31.11,26.85 C7.2 | 62.5,35.2 67.3,35.2 68.1,34.4 71.3,34.4 71.48,34.58 71.48,35.29 72.99,36.8 72.99,40.8 74.77,42.58 74.77,50.67 R7.2 | IC1.1 55.12,32.36 55.56,31.91 55.56,30.67 54.76,29.87 54.5,29.87 IC1.3 54.32,29.78 54.05,29.78 53.34,29.07 53.34,28.09 54.23,27.2 54.67,27.2 55.38,26.49 55.38,24.15 | 35.92,22.14 35.92,18.22 36.18,17.96 48.45,17.96 52.18,21.69 52.18,23.91 52,24 | 43,31.5 43.12,31.38 43.65,31.38 49.61,25.43 49.61,24.18 49.65,24 | 49.2,43.7 49.78,43.12 49.78,36.63 49.34,36.18 49.25,36
  Top 0.406: C11.1 C13.1 C12.1 33.65,49 36.5,49 | 36.5,49 36.88,48.62 U$2.GND 36.88,45.88 35.86,44.86 C2.2 | C10.1 C9.1 45.65,37.85 47.5,36 49.25,36 52.75,32.5 54.34,32.5 | U1.5 41.35,38.4 41.5,38.25 41.5,37 | 41.5,37 41.25,36.75 40.34,36.75 U1.3 | 54.34,32.5 IC1.1 | U1.21 arc-90 31.61,37.5 30,37.5 arc90 29.73,37.23 RST.2 arc-90 30,30.73 30,27 arc90 30.15,26.85 C7.2 | U2.2 41.5,28 arc-90 41,28.5 41,30 41.5,30 43,31.5 43,36 42,37 41.5,37 | Q3.2 61.95,41.5 61,41.5 60.35,42.15 R10.2 R12.2 60.85,37.5 61.5,37.5 62.5,36.5 62.5,35.2 62.5,34.5 61.5,33.5 56,33.5 55,32.5 54.34,32.5 | Q1.6 48.53,53.62 arc45 48.29,54.21 arc45 47.59,54.5 46,54.5 | 46,54.5 42.41,54.5 arc45 41.71,54.21 36.5,49 | J2.6 36.21,53.25 arc-45 36.5,52.55 36.5,49 | C5.2 49.65,24 52,24 52.15,24.15 R1.2 55.38,24.15 C1.2 | Q2.2 56.45,49.45 52,45 R4.2 49.5,44.65 49.5,44 49.2,43.7 49,43.5 46.5,43.5 46,44 46,54.5 | Q4.2 25.05,23.45 24,24.5 24,25.09 U$1.1 | C8.2 18.5,32.35 18.5,37 19.5,38 19.85,38 arc-90 R13.2 R11.1 18.8,42.15 arc-90 Q5.2
  Top 0.508: v32,22 32.15,22.15 C6.2
  Bottom 0.305: v32,25.96 32,22.05 v32,22
  other vias: 49,27 61,9.5 54.5,6.5 30,4.5 20.5,8.5 8.5,21 4.5,30 4,48 8,58 18.5,70.5 29,75.5 54.5,74 60.5,70.5 69.5,62 73.5,56.5 76.5,32
  pour Top: -16,89 91,87 91,-3 -16,-3
  pour Bottom: -10,90 91,93.5 91,-6 -10,-8
GND-ISO
  Top 0.305: Q1.2 49.19,57.23 arc45 49.48,56.52 51,55 51,49.29 arc-45 50.71,48.59 IC2.6
  Top 0.406: C4.1 arc-90 48.53,61.12 Q1.3 Q1.2
  Top 0.61: C4.1 37.5,61.5 arc-90 35,64 35,76.57 arc90 BT2.-
N$1
  Top 0.406: Q1.5 47.91,52.64 IC2.3
N$2
  Top 0.406: BLUE.C R7.1
N$3
  Top 0.406: IC1.2 53.53,31.11 arc45 52.82,30.82 52.79,30.79 arc45 52.5,30.09 52.5,27.91 arc45 52.79,27.21 54.15,25.85 R1.1
N$4
  Top 0.406: GREEN.C R2.1
N$5
  Top 0.406: RED.C R3.1
N$6  (via drill 0.35)
  Top 0.203: v61.25,30.85 60.27,29.87 59.92,29.87 IC1.6 | v58.23,27.91 58.5,27.91 58.56,27.85 arc45 59.27,27.56 62.7,27.56 arc45 63.41,27.85 64.45,28.89 64.5,29
  Top 0.254: R2.2 70.79,25.32 arc-45 70.5,26.02 70.5,28.09 arc45 70.21,28.79 68.79,30.21 arc45 68.09,30.5 66.41,30.5 arc45 65.71,30.21 64.5,29
  Bottom 0.203: v61.25,30.85 58.32,27.91 v58.23,27.91
N$7  (via drill 0.35)
  Top 0.203: v46.94,17.07 47.77,17.07 arc45 48.48,17.36 51.71,20.6 arc-45 52.42,20.89 62.53,20.89 arc45 63.23,21.18 65.08,23.02 65.08,23.11 65.16,23.2 65.16,23.38 65.25,23.47 65.25,23.56 65.34,23.65 65.34,23.74 65.43,23.82 65.43,24 65.61,24.18 70.08,24.18 arc-45 70.79,23.89 71.74,22.94 71.83,22.94 71.92,22.85 72.1,22.85 72.19,22.76 72.28,22.76 72.36,22.67 72.45,22.67 72.54,22.58 72.72,22.58 72.81,22.49 72.9,22.49 73.17,22.76 arc-45 73.29,23.06 73.85,23.62 arc45 74.14,24.33 74.14,27.2 R3.2 | v58.32,32.72 58.66,32.37 arc-45 58.85,31.91 59.65,31.11 IC1.7
  Bottom 0.203: v58.32,32.72 47.23,21.63 arc45 46.94,20.92 v46.94,17.07
N$8
  Top 0.406: IC2.2 48.86,49.45 arc-45 48.79,49.29 arc-45 48.09,49 48,49 arc90 47,48 47,46.56 arc45 47.29,45.86 R4.1
N$9
  Top 0.305: IC2.5 48.86,47.5 arc90 49.86,46.5 50.44,46.5 arc45 51.14,46.79 R5.1
N$10
  Top 0.203: C9.2 44.54,36.01 44.54,35.2 48.45,31.29 Y1.2
  Top 0.305: U1.7 41.5,40 arc-90 42.25,39.5 42.25,37.75 43.85,36.15 C9.2 | Y1.2 48.5,31.15
N$11
  Top 0.305: U1.8 arc-90 41.34,41.85 C10.2 46.98,41.85 arc-90 Y1.1
N$12
  Top 0.406: U2.1 arc-90 42.3,29 43.5,29 43.5,23.18 arc-90 L2.1
  Top 0.508: L2.1 40.07,19.74 arc-45 39.36,19.45 D1.2
N$13
  Top 0.406: U2.3 42.2,27 R8.2 R9.1
N$14  (via drill 0.35)
  Top 0.406: U2.5 U2.4 | S1.2 77.5,40 78.21,40.71 arc45 78.5,41.41 78.5,45.34 arc18 78.45,45.65 77.55,48.35 arc-18 77.5,48.66 77.5,50.61 arc45 77.21,51.32 BLUE.A | v51.5,22 arc-90 51,21.5 48.85,21.5
  Top 0.508: C5.1 48.85,21.5 L2.2 46.12,25.26 arc45 45.83,25.97 U2.4
  Bottom 0.508: S1.2 76.5,40 72.79,36.29 arc-45 72.09,36 67.41,36 arc45 66.71,35.71 65.79,34.79 arc45 65.5,34.09 65.5,32.41 arc-45 65.21,31.71 63.29,29.79 arc45 63,29.09 arc-45 62.94,28.94 56.29,22.29 arc-45 55.59,22 v51.5,22
N$15
  Top 0.406: R10.1 59.65,43.5 58.91,43.5 arc45 58.21,43.21 58.04,43.04 arc-45 57.34,42.75 IC4.3
N$16
  Top 0.305: R14.1 D2.A
N$17
  Top 0.305: R11.2 20,44 arc-90 20.5,44.5 24.5,44.5 arc-108 IC3.3
N$18
  Top 0.305: R15.1 D3.A
N$19
  Top 0.305: R16.1 60.35,60.2 D4.A
N$20
  Top 0.305: R17.1 D5.A
N$21
  Top 0.305: D6.A 68.9,39.83 R18.1
N$22
  Top 0.305: R19.1 D7.A
N$23
  Top 0.305: R20.1 D8.A
N$24
  Top 0.305: R21.1 D9.A
N$25
  Top 0.305: R22.1 D10.A
N$26
  Top 0.305: R23.1 D11.A
N$27
  Top 0.305: R26.1 D14.A
N$28
  Top 0.305: R25.1 D13.A
N$29
  Top 0.305: R24.1 D12.A
N$30
  Top 0.305: R27.1 D15.A
N$31
  Top 0.305: R28.1 D16.A
N$32
  Top 0.305: R29.1 D17.A
N$34
  Top 0.406: D4.K arc90 61.8,62.5 58.5,62.5 arc90 55.5,59.5 Q2.3
  Bottom 0.406: D2.K D3.K D4.K D5.K
N$35
  Top 0.305: D6.K arc90 68.77,42.5 Q3.3
  Bottom 0.203: 61.11,28.39 63.27,30.55 arc45 63.56,31.26 63.56,32.92 arc-45 63.86,33.63 66.58,36.35 arc-45 67.03,36.54 70.41,39.92 71.21,39.92 D6.K | 60.98,28.27 61.11,28.39 | 61.11,28.39 55.29,22.94 arc-43 54.6,22.67 51.21,22.67 50.85,22.31 50.85,21.75 arc45 51.14,21.04 57.34,14.85 57.45,14.68
  Bottom 0.406: D7.K D8.K 57.45,14.68 D9.K
N$36
  Top 0.406: Q4.3 24.17,18.57 arc-45 24,18.5 arc-45 22.44,17.85 D12.K
  Bottom 0.406: D13.K D12.K D11.K D10.K
N$37
  Top 0.305: Q5.3 15.9,44.6 arc90 13,47.5 arc-90 11,49.5 arc-12 D15.K
  Bottom 0.406: D14.K D15.K D16.K D17.K
N$38
  Top 0.406: Q2.1 54.55,54.4 R30.2
N$39
  Top 0.406: Q3.1 62.71,42.74 arc-45 63,42.04 63,40.91 arc45 63.29,40.21 63.85,39.65 R31.2
N$40
  Top 0.305: R32.2 27.94,22.21 arc45 27.24,22.5 Q4.1
N$41
  Top 0.406: Q5.1 17.55,41.05 16.5,40 16.5,39.35 R33.2
OD
  Top 0.305: IC2.1 50.5,50.88 50.5,54.5 48.18,56.82 arc-45 47.88,57.53 Q1.4
RESET
  Top 0.254: U1.29 36.4,31.55 C3.2 34.15,29.3 R6.1 32.27,30.88 RST.1
  Top 0.305: U1.29 arc-90 36.5,33.61
RESET_CAP  (via drill 0.35)
  Top 0.203: v34,32.1 34.08,31.93 34.08,31.07
  Top 0.254: v33.5,36 33.06,35.56 arc45 33,35.41 arc-45 32.71,34.71 32.29,34.29 arc45 32,33.59 32,33.41 arc45 32.29,32.71 32.5,32.5 arc-45 32.76,32.39 34.08,31.07 C3.1
  Bottom 0.203: J1.D- 40.65,5.65 arc-90 41.5,6.5 42.5,6.5 44,8 44,24.59 arc45 43.71,25.29 37.29,31.8 arc45 36.58,32.1 v34,32.1
  Bottom 0.254: v33.5,36 31.5,36 28.79,38.71 arc-45 28.5,39.41 28.5,41.59 arc45 28.21,42.29 23.29,47.21 arc-45 23,47.91 J2.1
RXD  (via drill 0.35)
  Top 0.203: U1.30 37.2,33.21 arc45 37.49,32.51 v38.5,31.5 | v42.5,13.5 44,15 v45.5,15
  Top 0.254: U1.30 37.25,33.76 37.25,35.59 arc45 36.96,36.29 36.54,36.71 arc45 35.84,37 v33.5,37
  Bottom 0.203: 39.5,4.83 J1.ID 39.35,5.94 arc-45 39.64,6.64 40.07,7.07 arc-45 40.5,7.25 arc-45 41.1,7.5 41.34,7.5 arc45 42.04,7.79 42.71,8.46 arc45 43,9.16 43,13 v42.5,13.5 | v38.5,31.5 44.21,25.79 arc-45 44.5,25.09 44.5,16 v45.5,15
  Bottom 0.254: v33.5,37 32,37 29.29,39.71 arc-45 29,40.41 29,42.09 arc45 28.71,42.79 25.29,46.21 arc-45 25,46.91 25,50.09 J2.2
TXD  (via drill 0.35)
  Top 0.203: v45.5,17 44.5,17 v43,15.5
  Top 0.254: v33.5,38 36.09,38 arc-45 36.79,37.71 37.46,37.04 arc-45 37.75,36.34 37.75,35.35 arc45 38,34.75 U1.31 38,33.41 arc45 38.29,32.71 v38.5,32.5
  Bottom 0.203: J1.D+ 40,5.59 arc-45 40.29,6.29 40.71,6.71 arc-45 41.41,7 41.59,7 arc45 42.29,7.29 43.21,8.21 arc45 43.5,8.91 43.5,15.5 v43,15.5 | 39,32.5 44.71,26.79 arc-45 45,26.09 45,17.5 v45.5,17
  Bottom 0.254: J2.3 26.5,52 26.5,46.41 arc45 26.79,45.71 29.71,42.79 arc-45 30,42.09 30,40.41 arc45 30.29,39.71 32,38 v33.5,38 | v38.5,32.5 39,32.5
V_BATT  (via drill 0.35)
  Top 0.406: v54.5,50 52.65,50 R5.2
  Top 0.508: IC1.5 61.66,28.57 arc45 62.37,28.87 66.21,32.71 arc-45 66.91,33 72.09,33 arc45 72.79,33.29 74.71,35.21 arc45 75,35.91 75,41 arc-90 76,42 S1.1
  Top 0.61: 52.65,50 52.65,55.85 51,57.5 51,59.94 arc45 50.71,60.64 C4.2 49.85,62 arc90 48.85,63 48.5,63 arc-90 47.5,64 47.5,75.6 arc90 46.5,76.6 BT2.+
  Bottom 0.61: S1.1 v54.5,50
VIN  (via drill 0.35)
  Top 0.406: IC1.4 arc90 55.53,27.5 56,27.5 arc-90 57,26.5 | 57,26.5 C1.1 | GREEN.A v75.31,24.61 RED.A | IC1.8 62.12,32.38 v62.5,32 64,32 66.5,34.5 v67,34.5 | v58.5,27 57.5,27 57,26.5
  Bottom 0.406: v58.5,27 62.21,30.71 arc45 62.5,31.41 v62.5,32 | v67,34.5 67.5,34.5 71.71,30.29 arc-45 72,29.59 72,26.41 arc45 72.29,25.71 73.1,24.9 arc45 73.81,24.61 v75.31,24.61
  Bottom 0.508: J1.VBUS 41.3,5.8 42.39,5.8 arc45 43.09,6.09 46.71,9.71 arc45 47,10.41 47,16 49,18 49,21.09 arc-45 49.29,21.79 51.71,24.21 arc-45 52.41,24.5 56,24.5 v58.5,27

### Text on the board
tPlace: iO Athlete
228bmp: ©nearIO 2019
